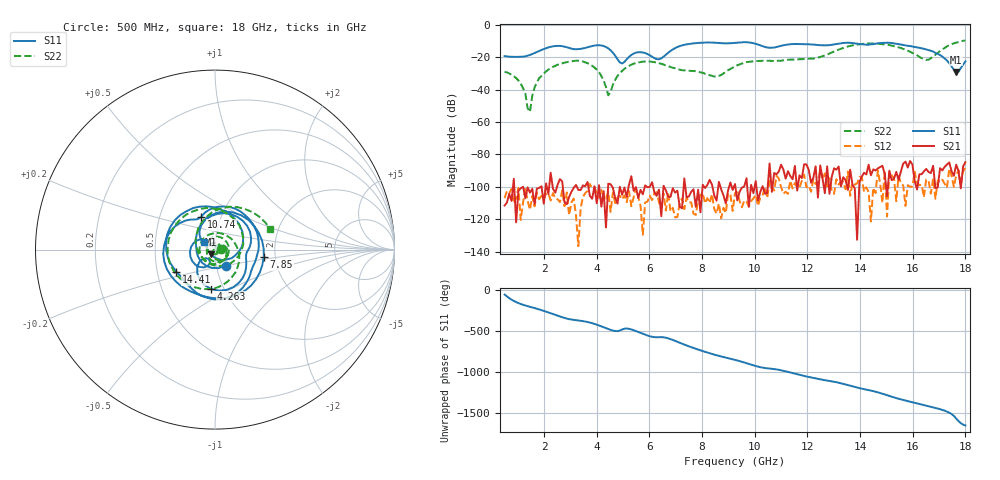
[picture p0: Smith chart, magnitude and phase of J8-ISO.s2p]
!Agilent Technologies,N5230A,MY45001360,A.07.50.67
!Agilent N5230A: A.07.50.67
!Date: Tuesday, April 16, 2024 16:04:51
!Correction: S11(Full 2 Port(1,2))
!S21(Full 2 Port(1,2))
!S12(Full 2 Port(1,2))
!S22(Full 2 Port(1,2))
!S2P File: Measurements: S11, S21, S12, S22:
# Hz S  dB  R 50
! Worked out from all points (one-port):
!   201 points, 500 MHz to 18 GHz, reference 50 ohm
!   lowest |S11| = -29.1 dB at 17.65 GHz (marker M1), VSWR 1.07, Z = 47.7 - j2.55 ohm
!   |S11| at or under -10 dB: start of sweep to end of sweep
!   S11 on the Smith chart (normalised r, x): 500 MHz: 1.11, -0.20; 4.263 GHz: 0.87, -0.40; 7.85 GHz: 1.74, -0.15; 10.74 GHz: 0.81, +0.31; 14.41 GHz: 0.63, -0.17; 18 GHz: 0.88, +0.08
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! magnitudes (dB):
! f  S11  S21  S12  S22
! 500 MHz  -19.3  -111.5  -106.9  -29.0
! 1.113 GHz  -19.8  -100.8  -120.4  -36.3
! 1.462 GHz  -18.7  -103.5  -114.1  -53.7
! 1.637 GHz  -17.5  -110.7  -112.0  -38.7
! 1.988 GHz  -15.0  -110.3  -107.6  -30.1
! 3.475 GHz  -14.6  -99.1  -106.2  -22.7
! 4.263 GHz  -13.1  -102.6  -106.4  -34.4
! 4.438 GHz  -14.6  -98.0  -103.0  -43.5
! 4.875 GHz  -23.2  -100.0  -105.4  -29.8
! 5.138 GHz  -21.3  -106.0  -109.4  -26.2
! 5.662 GHz  -16.9  -101.8  -111.7  -23.0
! 6.362 GHz  -21.3  -101.6  -109.5  -23.7
! 7.85 GHz  -11.2  -101.7  -108.2  -28.9
! 8.55 GHz  -11.2  -108.5  -116.4  -31.8
! 9.25 GHz  -11.1  -98.2  -103.8  -25.7
! 10.74 GHz  -14.1  -91.4  -102.3  -22.4
! 12.22 GHz  -12.2  -94.3  -95.3  -20.9
! 14.41 GHz  -12.1  -92.8  -121.3  -11.6
! 15.11 GHz  -11.1  -89.9  -90.8  -12.5
! 16.51 GHz  -15.2  -88.9  -95.4  -21.6
! 17.65 GHz  -29.1  -86.3  -92.7  -11.0
! 18 GHz  -22.6  -84.7  -88.4  -9.7
